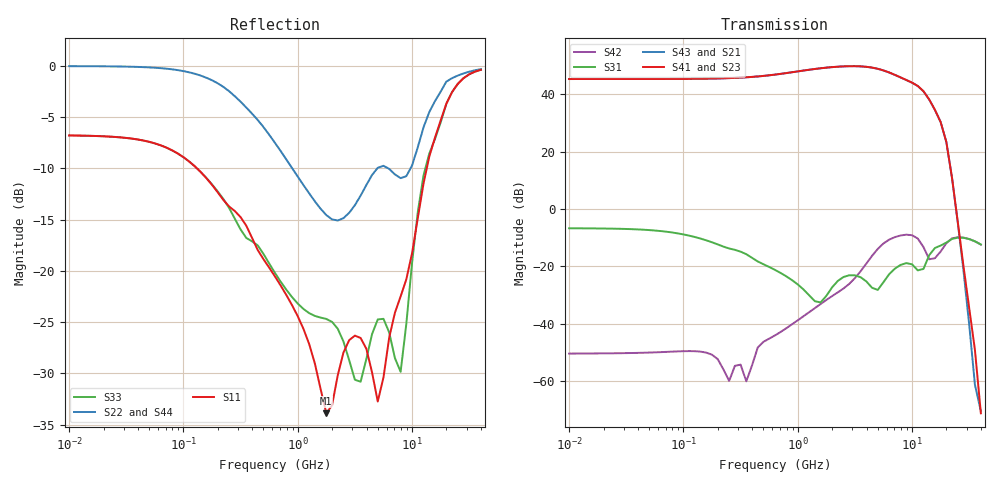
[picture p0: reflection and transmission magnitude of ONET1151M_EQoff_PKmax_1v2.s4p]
! Touchstone Ver. 1.0
! Thu Sep  6 15:55:40 2012
! Number of ports is 4
# Hz	S	DB	R	50.000000
! SCATTERING PARAMETERS  :
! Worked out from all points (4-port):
!   73 points, 10 MHz to 40 GHz, reference 50 ohm
!   strongest paths, dB at 10 MHz, 79.43 MHz, 631 MHz, 5.012 GHz, 40 GHz:
!     S41: 45.2, 45.3, 46.8, 48.8, -71.2
!     S43: 45.3, 45.3, 46.8, 48.8, -70.5
!     S21: 45.3, 45.3, 46.8, 48.9, -70.1
!     S23: 45.3, 45.3, 46.8, 48.9, -70.6
!     S31: -6.7, -8.2, -21.2, -28.2, -12.4
!     S42: -50.4, -49.7, -44.1, -13.9, -12.4
!   lowest |S11| = -33.9 dB at 1.778 GHz (marker M1), VSWR 1.04, Z = 51.1 - j1.72 ohm
!   |S11| at or under -10 dB: 131.2 MHz to 13.47 GHz (13.34 GHz wide, 196 % of centre)
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1e7  -6.80 -4.5  -110.52 176.9  -6.73 -4.3  -110.49 176.9
     45.26 -175.5  -0.05 7.1  45.26 4.5  -50.47 9.5
     -6.73 -4.3  -110.51 176.8  -6.80 -4.5  -110.51 176.9
     45.25 4.5  -50.37 9.5  45.25 -175.5  -0.05 7.1
1.778279e9  -33.88 -56.1  -39.35 56.9  -26.46 -47.6  -39.28 57.0
            49.26 116.2  -14.56 -84.7  49.26 -63.8  -34.67 24.8
            -30.27 8.7  -39.31 57.0  -24.69 -77.2  -39.28 56.9
            49.22 -64.1  -31.70 11.6  49.21 115.9  -14.40 -82.0
3.981072e9  -27.59 -87.6  -38.65 -7.7  -29.32 56.4  -38.59 -7.5
            49.59 9.1  -11.64 -111.1  49.58 -170.9  -18.61 -121.5
            -25.23 -69.2  -38.62 -7.4  -28.60 88.9  -38.58 -7.7
            49.52 -171.6  -19.02 -125.8  49.50 8.4  -11.87 -112.7
5.623413e9  -30.38 109.7  -37.43 -29.4  -30.91 17.1  -37.38 -29.1
            48.39 -68.2  -9.76 -164.6  48.37 111.8  -11.53 161.5
            -25.49 142.7  -37.41 -29.0  -24.67 3.7  -37.37 -29.4
            48.25 111.2  -12.01 160.8  48.24 -68.8  -10.10 -163.9
7.943282e9  -22.49 33.6  -38.18 -64.9  -23.15 89.2  -38.16 -64.4
            45.95 -169.9  -10.97 136.4  45.93 10.2  -9.08 90.2
            -19.48 73.2  -38.19 -64.3  -29.84 16.0  -38.10 -64.9
            45.82 9.7  -9.23 91.4  45.79 -170.2  -10.90 137.6
1e10  -18.28 27.4  -39.56 -88.5  -19.18 64.1  -39.57 -87.7
      44.12 101.4  -9.73 99.6  44.10 -78.4  -9.22 47.7
      -19.28 45.6  -39.62 -87.4  -19.21 44.8  -39.48 -88.7
      44.00 -79.0  -9.14 48.1  43.97 101.1  -9.59 98.5
4e10  -0.40 -143.6  -68.63 142.1  -12.37 -52.7  -68.44 141.9
      -70.10 -145.8  -0.33 -143.9  -70.56 58.4  -12.41 -53.3
      -12.37 -52.7  -68.36 141.6  -0.40 -143.5  -68.62 142.3
      -71.17 60.8  -12.41 -53.3  -70.48 -145.0  -0.33 -143.9
